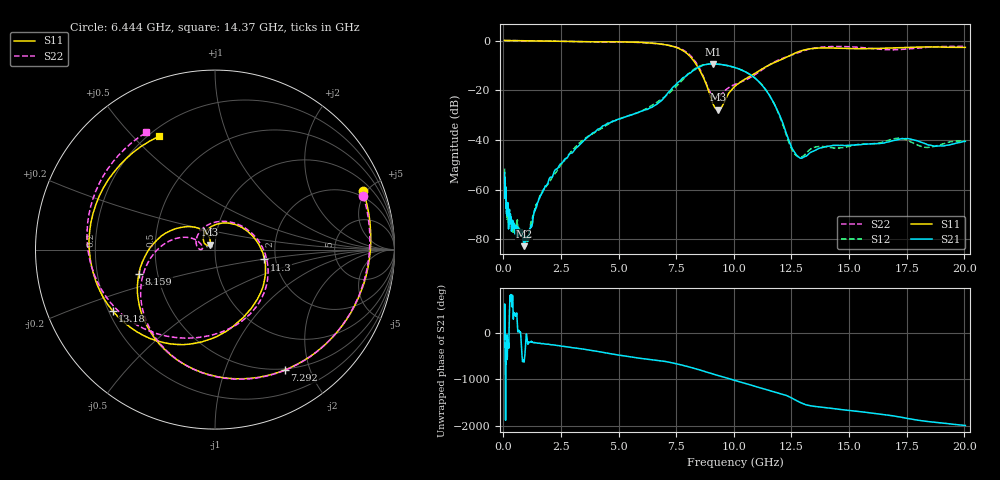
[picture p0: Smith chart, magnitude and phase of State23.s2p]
# Hz S DB R 50
!freq MagS11 AngS11 MagS21 AngS21 MagS12 AngS12 MagS22 AngS22
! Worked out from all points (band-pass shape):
!   1601 points, 50 MHz to 20.05 GHz, reference 50 ohm
!   highest |S21| = -9.41 dB at 9.095 GHz (marker M1); lowest = -82.8 dB at 888.1 MHz (marker M2)
!   |S21| within 3 dB of the highest: 8.189 GHz to 10.46 GHz (2.272 GHz wide, 24.4 % of centre)
!   lowest |S11| = -27.8 dB at 9.302 GHz (marker M3), VSWR 1.08, Z = 47 + j2.62 ohm
!   |S11| at or under -10 dB: 8.393 GHz to 11.51 GHz (3.112 GHz wide, 31.3 % of centre)
!   |S22| runs from -23.1 to 0.0 dB; largest |S21 - S12| = 0.021
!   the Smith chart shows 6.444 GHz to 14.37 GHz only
!   S11 on the Smith chart (normalised r, x): 6.444 GHz: 1.56, +4.79; 7.292 GHz: 0.48, -1.63; 8.159 GHz: 0.39, -0.13; 11.3 GHz: 1.74, -0.21; 13.18 GHz: 0.22, -0.26; 14.37 GHz: 0.24, +0.59
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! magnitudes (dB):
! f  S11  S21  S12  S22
! 50 MHz  0.0  -53.2  -51.5  0.0
! 56.37 MHz  0.0  -62.6  -56.5  0.0
! 63.79 MHz  0.0  -56.1  -57.8  0.0
! 135.9 MHz  0.0  -69.7  -66.8  0.0
! 193.3 MHz  0.0  -66.1  -71.8  0.0
! 221.2 MHz  0.0  -75.8  -73.1  0.0
! 255.1 MHz  0.0  -68.5  -71.1  0.0
! 369.6 MHz  0.0  -75.7  -75.0  0.0
! 888.1 MHz  -0.1  -82.8  -78.6  -0.1
! 1.005 GHz  -0.1  -80.0  -80.9  -0.1
! 2.722 GHz  -0.3  -47.5  -47.3  -0.4
! 6.444 GHz  -1.0  -26.9  -26.0  -1.1
! 7.292 GHz  -2.2  -19.5  -20.3  -2.2
! 7.402 GHz  -2.5  -18.4  -19.3  -2.4
! 8.159 GHz  -7.0  -12.7  -12.4  -6.5
! 9.095 GHz  -25.5  -9.4  -9.4  -22.5
! 9.302 GHz  -27.8  -9.5  -9.5  -22.9
! 11.3 GHz  -11.0  -18.9  -18.7  -11.3
! 12.6 GHz  -5.3  -44.5  -45.1  -5.5
! 13.18 GHz  -3.6  -46.3  -45.0  -3.7
! 14.37 GHz  -3.0  -42.2  -43.3  -2.4
! 20.05 GHz  -2.8  -40.6  -40.4  -2.4
